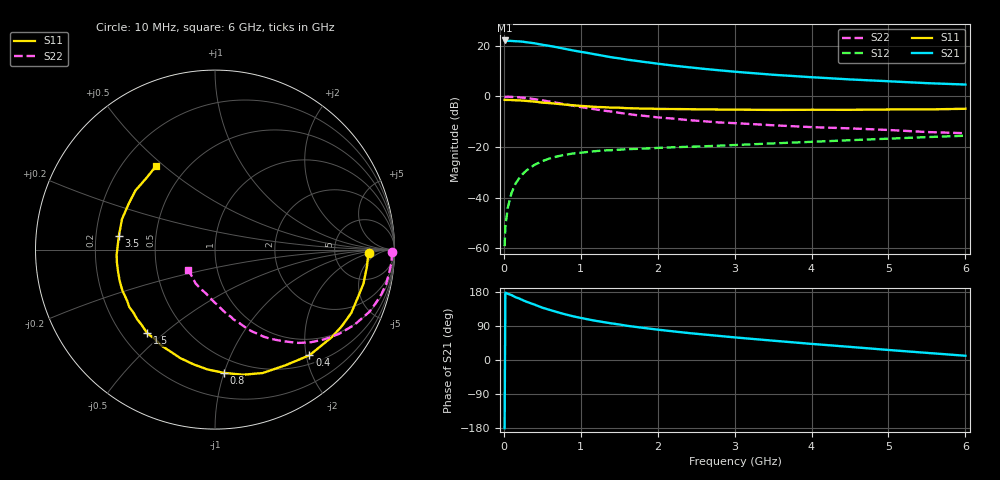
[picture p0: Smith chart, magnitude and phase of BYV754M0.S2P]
! SIEMENS Small Signal Semiconductors
! BFY420
! Si NPN RF SIEGET Grounded Emitter Transistor in MICRO-X
! VCE = 0.75 V  IC = 4 mA
! Common Emitter S-Parameters:  October  1996
# GHz  S  MA  R  50
!  f  S11  S21  S12  S22
! GHz  MAG  ANG  MAG  ANG  MAG  ANG  MAG  ANG
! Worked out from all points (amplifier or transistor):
!   36 points, 10 MHz to 6 GHz, reference 50 ohm
!   highest |S21| = 22.1 dB at 10 MHz (marker M1)
!   |S21| within 3 dB of that: start of sweep to 742.5 MHz
!   unconditionally stable (mu >= 1): 3.25 GHz to end of sweep
!   at 250 MHz: K = 0.10, MSG = 26.1 dB, |S12| = -30.5 dB
!   at 1.4 GHz: K = 0.49, MSG = 18.3 dB, |S12| = -21.2 dB
!   at 6 GHz: K = 1.19, MAG = 7.5 dB, |S12| = -15.5 dB
!   S11 on the Smith chart (normalised r, x): 10 MHz: 13, -2; 400 MHz: 0.66, -2.06; 800 MHz: 0.38, -1.00; 1.5 GHz: 0.30, -0.44; 3.5 GHz: 0.30, +0.07; 6 GHz: 0.34, +0.47
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0.01  0.8558 -1.3  12.77 -179.9  0.0011 104.1  0.9873 -0.8
0.02  0.8532 -2.7  12.71 177.8  0.0027 90.9  0.9832 -1.4
0.05  0.8519 -6.3  12.53 174.9  0.0062 88.0  0.987 -3.7
0.1  0.8487 -12.9  12.49 171.3  0.0124 83.7  0.9788 -7.6
0.15  0.8392 -18.7  12.33 165.9  0.0188 78.7  0.9726 -11.3
0.2  0.8373 -25.0  12.23 162.3  0.0242 76.8  0.9604 -14.9
0.3  0.8134 -36.8  11.74 153.3  0.0351 69.9  0.9279 -21.9
0.4  0.7897 -48.2  11.21 146.1  0.0446 64.4  0.883 -28.3
0.5  0.7547 -58.6  10.5 138.1  0.0527 59.1  0.8364 -34.1
0.6  0.7372 -68.9  9.921 132.0  0.0598 54.4  0.7888 -39.3
0.8  0.6881 -86.0  8.677 120.4  0.0704 46.8  0.6976 -48.2
0.9  0.6689 -93.6  8.106 115.3  0.0745 43.7  0.6555 -51.6
1.1  0.6345 -107.8  7.187 107.0  0.0804 38.8  0.5834 -58.3
1.3  0.613 -118.9  6.324 99.9  0.0856 35.1  0.5243 -63.3
1.5  0.5994 -129.1  5.663 93.8  0.0885 32.3  0.4753 -67.8
1.8  0.5744 -142.3  4.854 85.1  0.093 29.8  0.4166 -73.2
2.2  0.5644 -156.0  4.065 75.6  0.0989 27.0  0.3648 -79.6
2.8  0.5513 -172.4  3.285 63.5  0.1065 25.0  0.3059 -87.9
3.5  0.5411 171.8  2.682 51.0  0.1181 22.9  0.2693 -96.1
4.5  0.5442 152.6  2.168 34.6  0.1364 19.0  0.2337 -109.5
5.5  0.5527 133.3  1.83 18.8  0.1573 13.9  0.1979 -129.8
6  0.5708 125.0  1.717 11.2  0.1674 10.7  0.1875 -142.4
